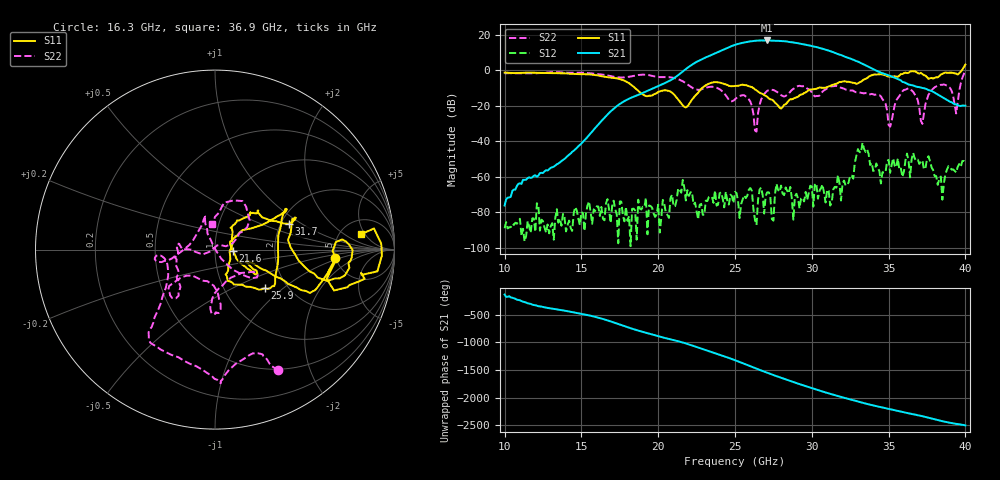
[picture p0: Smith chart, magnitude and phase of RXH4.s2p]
!Keysight Technologies,M9808A,MY58100618,A.14.70.03
!Date: Monday, February 27, 2023 13:24:57
!Correction: S11(Cdelta 2-Port  )
!S21(Cdelta 2-Port  )
!S12(Cdelta 2-Port  )
!S22(Cdelta 2-Port  )
!S2P File: Measurements: S11, S21, S12, S22:
# Hz S  RI  R 50
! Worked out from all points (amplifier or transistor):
!   301 points, 10 GHz to 40 GHz, reference 50 ohm
!   highest |S21| = 16.7 dB at 27.1 GHz (marker M1)
!   |S21| within 3 dB of that: 24.83 GHz to 29.93 GHz (5.1 GHz wide, 18.6 % of centre)
!   unconditionally stable (mu >= 1): start of sweep to 39.73 GHz
!   at 15 GHz: K = 70124.98, MAG = -32.1 dB, |S12| = -80.0 dB
!   at 25 GHz: K = 225.76, MAG = 14.9 dB, |S12| = -68.7 dB
!   at 40 GHz: K = 2.89, MSG = 15.8 dB, |S12| = -51.6 dB
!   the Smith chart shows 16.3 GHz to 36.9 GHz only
!   S11 on the Smith chart (normalised r, x): 16.3 GHz: 4.96, -0.83; 21.6 GHz: 1.22, -0.02; 25.9 GHz: 1.54, -0.76; 31.7 GHz: 2.20, +0.78; 36.9 GHz: 7.89, +4.08
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1e10  -0.000743 0.851  -0.000104 -0.000113  1.49e-05 -3.17e-05  0.7464 0.337
1.5e10  0.7379 0.2038  -0.00455 -0.00724  7.89e-05 6.12e-05  0.6128 -0.5791
1.63e10  0.671 -0.0457  -0.0326 0.0168  -9.69e-05 -0.000102  0.3537 -0.6692
2e10  0.2148 -0.1115  -0.3499 -0.0695  3.65e-05 0.000158  -0.1704 -0.6206
2.16e10  0.1011 -0.00676  0.1956 0.893  -0.000228 -0.000777  -0.3278 -0.3588
2.28e10  0.2621 0.1374  1.673 -1.086  3.06e-05 -0.000168  -0.2832 -0.0467
2.37e10  0.4002 0.2252  -1.334 -2.639  0.000401 -3.65e-05  -0.3249 -0.0655
2.45e10  0.3633 0.1166  -4.122 0.8461  0.000193 6.56e-05  -0.1694 0.00377
2.5e10  0.3511 -0.0708  -2.274 4.587  -0.000225 0.000292  -0.0762 0.1307
2.59e10  0.2773 -0.215  6.003 2.078  -0.000359 0.000233  -0.0529 0.1412
2.66e10  0.1254 -0.195  3.557 -5.828  -0.00028 -0.000326  0.066 -0.0809
2.71e10  0.0689 -0.1625  -2.496 -6.361  -0.000358 -5.67e-05  0.2069 -0.16
2.78e10  0.0855 -0.0538  -6.67 0.3176  -0.000426 1.3e-05  0.1952 -0.1253
2.86e10  0.0937 0.1182  -0.8329 6.108  0.000217 0.000465  -0.0048 -0.2467
2.94e10  0.133 0.1619  4.902 2.209  0.000253 3.34e-05  0.00275 -0.3504
3e10  0.1961 0.2066  4.128 -2.346  9.91e-05 -0.000522  0.0146 -0.2379
3.07e10  0.2398 0.2069  -0.1082 -3.991  -0.000297 -0.000522  -0.192 -0.1579
3.17e10  0.4099 0.1436  -2.804 -0.3357  -0.000923 -0.000589  -0.2177 -0.2715
3.27e10  0.4246 0.116  -0.636 1.858  -0.000611 -0.00063  -0.2139 -0.1518
3.5e10  0.6549 -0.00776  0.4921 -0.5203  0.00264 -0.00135  -0.0267 -0.0106
3.69e10  0.8141 0.0852  -0.3184 -0.1038  0.000406 0.00298  -0.014 0.14
4e10  1.276 -0.6491  0.0967 0.0224  -0.00264 -4.08e-05  0.4658 -0.8858
